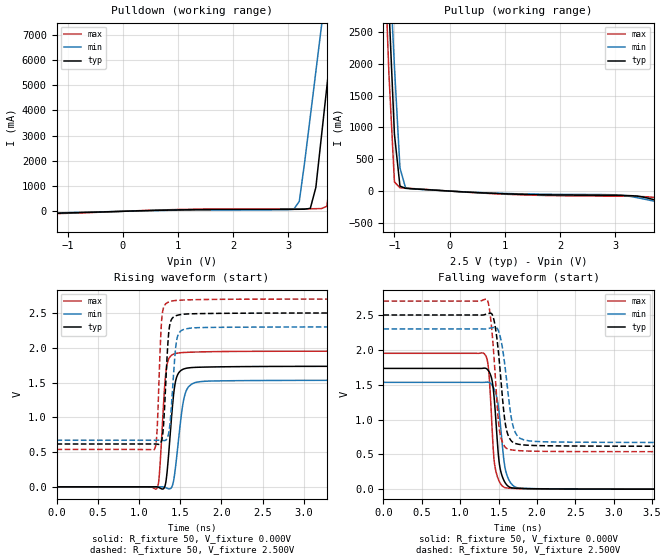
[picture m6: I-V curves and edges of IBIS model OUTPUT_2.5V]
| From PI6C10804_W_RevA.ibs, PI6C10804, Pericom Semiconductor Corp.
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[Model]   OUTPUT_2.5V
Model_type Output
Vref=2.500V
Vmeas=1.250V
| variable   typ   min   max
C_comp   1.150pF   1.149pF   1.151pF
[Voltage Range]   2.5000V   2.3000V   2.7000V
[POWER Clamp Reference]   2.5000V   2.3000V   2.7000V
[GND Clamp Reference]   0.0000V   0.0000V   0.0000V
[Pullup Reference]   2.5000V   2.3000V   2.7000V
[Pulldown Reference]   0.0000V   0.0000V   0.0000V
[Temperature Range]   25   85   -40
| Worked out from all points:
|   slope of the pulldown table from 0 to 0.375 V, typ, clamps not added: 15.4 ohm
|   slope of the pullup table from 0 to 0.375 V, typ, clamps not added: 20.1 ohm
|   falling waveform, R_fixture 50, V_fixture 0.000V: 20-80 % time 76.6ps typ, 92.5ps min, 63.5ps max; typ from 1.73 V to 0 V
|   rising waveform, R_fixture 50, V_fixture 0.000V: 20-80 % time 74.6ps typ, 92.6ps min, 59.5ps max; typ from 0 V to 1.73 V
|   falling waveform, R_fixture 50, V_fixture 2.500V: 20-80 % time 98.3ps typ, 113ps min, 85.1ps max; typ from 2.5 V to 0.616 V
|   rising waveform, R_fixture 50, V_fixture 2.500V: 20-80 % time 50.6ps typ, 60ps min, 42.5ps max; typ from 0.616 V to 2.5 V
[Pulldown]
| Voltage   I(typ)   I(min)   I(max)
-2.5V     -376.6mA   -306.4mA   -519.9mA
-1.2V     -78.61mA   -72.46mA   -92.58mA
3.1V      78.76mA    82.57mA    97.68mA
3.2V      80.55mA    393.4mA    98.12mA
3.4V      117.3mA    3.76A      100.8mA
3.5V      941.9mA    5.528A     103.3mA
3.6V      2.94A      7.296A     107.2mA
3.7V      4.937A     9.064A     199.3mA
3.8V      6.935A     10.83A     1.911A
4V        10.93A     14.37A     6.561A
4.1V      12.93A     16.14A     8.887A
5V        30.92A     32.06A     29.82A
[Pullup]
| Voltage   I(typ)   I(min)   I(max)
-2.5V     30.87A     28.49A     34.39A
-1.2V     4.887A     5.494A     4.164A
-1.1V     2.889A     3.725A     1.839A
-1V       890.5mA    1.956A     143.2mA
-900mV    78.6mA     362.9mA    52.61mA
-800mV    43.33mA    55.3mA     46.48mA
-700mV    37.46mA    35.65mA    40.95mA
1.2V      -48.17mA   -41.97mA   -55.85mA
3.1V      -67.89mA   -62.82mA   -80.61mA
3.4V      -78.07mA   -103.8mA   -84.36mA
3.7V      -134.2mA   -157.5mA   -98.86mA
5V        -448.1mA   -403.9mA   -535.9mA
[Falling Waveform]
R_fixture = 50
V_fixture = 0.000V
V_fixture_min = 0.000V
V_fixture_max = 0.000V
|   Time   V(typ)   V(min)   V(max)
0s        1.733V     1.533V     1.95V
1.32ns    1.737V     1.534V     1.935V
1.37ns    1.696V     1.534V     1.709V
1.415ns   1.559V     1.492V     875.3mV
1.45ns    1.203V     1.415V     342.9mV
1.51ns    361mV      1.066V     108.3mV
1.6ns     69.61mV    231mV      17.7mV
1.7ns     15.27mV    41.34mV    10.68mV
1.92ns    6.814mV    8.437mV    4.94mV
9.8ns     0V         1.248uV    0V
[Rising Waveform]
R_fixture = 50
V_fixture = 0.000V
V_fixture_min = 0.000V
V_fixture_max = 0.000V
|   Time   V(typ)   V(min)   V(max)
0s        0V         0V         0V
1.22ns    200.8uV    57.15uV    -20.42mV
1.25ns    -14.06mV   533.6uV    215.7mV
1.31ns    -6.371mV   -5.567mV   1.411V
1.335ns   142.1mV    -17.53mV   1.722V
1.405ns   1.137V     15.71mV    1.9V
1.45ns    1.546V     347.7mV    1.919V
1.56ns    1.701V     1.336V     1.933V
1.72ns    1.72V      1.509V     1.939V
8ns       1.733V     1.533V     1.95V
[Falling Waveform]
R_fixture = 50
V_fixture = 2.500V
V_fixture_min = 2.300V
V_fixture_max = 2.700V
|   Time   V(typ)   V(min)   V(max)
0s        2.5V       2.3V       2.7V
1.35ns    2.516V     2.302V     2.722V
1.39ns    2.525V     2.312V     2.509V
1.435ns   2.448V     2.321V     1.973V
1.51ns    1.825V     2.234V     856.1mV
1.58ns    995.9mV    1.791V     610.5mV
1.66ns    700.1mV    1.062V     565.7mV
1.76ns    644.5mV    746.4mV    553.2mV
2.02ns    625.1mV    683mV      544mV
9.8ns     616.1mV    669.9mV    538mV
[Rising Waveform]
R_fixture = 50
V_fixture = 2.500V
V_fixture_min = 2.300V
V_fixture_max = 2.700V
|   Time   V(typ)   V(min)   V(max)
0s        616.1mV    669.9mV    538mV
1.185ns   616.4mV    669.9mV    536.6mV
1.22ns    614.2mV    670.1mV    813.5mV
1.28ns    692.3mV    668.7mV    2.454V
1.3ns     918.6mV    666mV      2.582V
1.36ns    2.204V     767.4mV    2.657V
1.4ns     2.417V     1.267V     2.672V
1.465ns   2.466V     2.149V     2.682V
1.6ns     2.487V     2.278V     2.689V
8ns       2.5V       2.3V       2.7V
[Ramp]
| variable   typ   min   max
dV/dt_r   1.03812V/74.826p   0.91770V/92.674p   1.16850V/59.570p
dV/dt_f   1.13040V/98.102p   0.97722V/113.01p   1.29750V/85.165p
R_load = 50
